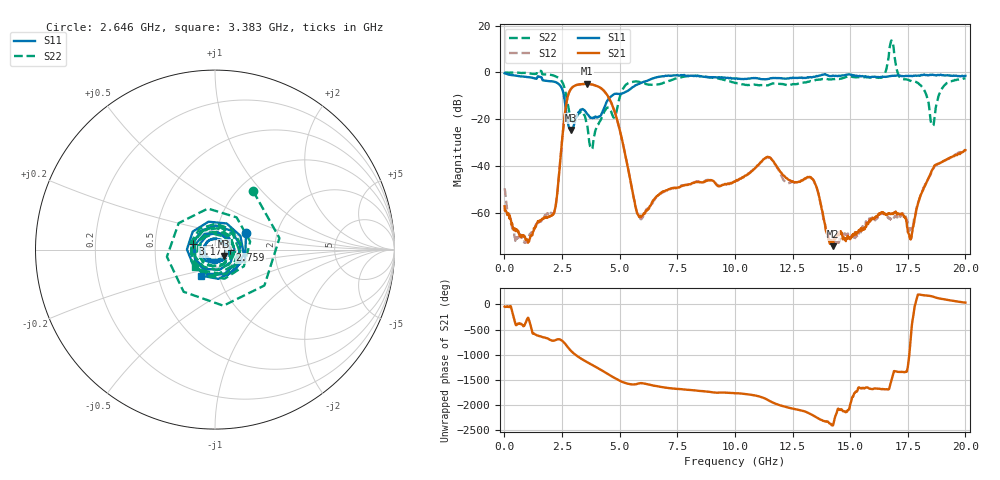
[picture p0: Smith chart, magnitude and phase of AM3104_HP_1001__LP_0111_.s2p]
!Created with skrf (http://scikit-rf.org).
# Hz S RI R 50.0
!freq ReS11 ImS11 ReS21 ImS21 ReS12 ImS12 ReS22 ImS22
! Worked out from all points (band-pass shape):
!   1601 points, 10 MHz to 20 GHz, reference 50 ohm
!   highest |S21| = -4.87 dB at 3.571 GHz (marker M1); lowest = -74.1 dB at 14.25 GHz (marker M2)
!   |S21| within 3 dB of the highest: 2.836 GHz to 4.32 GHz (1.484 GHz wide, 41.5 % of centre)
!   lowest |S11| = -24.6 dB at 2.884 GHz (marker M3), VSWR 1.13, Z = 54.9 - j3.83 ohm
!   |S11| at or under -10 dB: 2.583 GHz to 4.658 GHz (2.075 GHz wide, 57.3 % of centre)
!   |S22| runs from -32.6 to 13.6 dB; largest |S21 - S12| = 0.037
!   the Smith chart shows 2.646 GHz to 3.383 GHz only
!   S11 on the Smith chart (normalised r, x): 2.646 GHz: 1.39, +0.27; 2.759 GHz: 1.18, -0.01; 3.171 GHz: 0.78, +0.05; 3.383 GHz: 0.82, -0.24
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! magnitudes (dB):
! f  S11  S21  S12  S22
! 10 MHz  -0.3  -57.1  -49.4  0.0
! 884.6 MHz  -1.8  -70.1  -72.6  -0.2
! 2.121 GHz  -3.9  -60.6  -60.1  -1.3
! 2.646 GHz  -14.1  -16.0  -16.0  -8.2
! 2.759 GHz  -21.5  -10.0  -10.0  -13.9
! 2.884 GHz  -24.6  -7.1  -7.2  -19.9
! 3.171 GHz  -17.9  -5.3  -5.3  -18.1
! 3.346 GHz  -15.8  -5.0  -5.1  -16.5
! 3.383 GHz  -15.6  -5.0  -5.0  -16.7
! 3.571 GHz  -17.4  -4.9  -4.9  -21.8
! 3.771 GHz  -19.3  -5.1  -5.1  -31.9
! 4.695 GHz  -9.7  -14.3  -14.4  -18.5
! 5.845 GHz  -4.9  -61.7  -61.9  -4.0
! 6.682 GHz  -1.9  -52.4  -52.4  -5.1
! 10.01 GHz  -2.7  -46.6  -46.7  -4.5
! 11.44 GHz  -2.8  -36.1  -36.2  -5.5
! 13.34 GHz  -2.1  -45.3  -45.3  -3.7
! 14.25 GHz  -1.3  -74.1  -72.3  -2.9
! 16.68 GHz  -1.6  -60.5  -62.3  7.2
! 17.61 GHz  -1.5  -70.8  -66.5  -3.5
! 18.56 GHz  -0.9  -41.5  -41.8  -22.3
! 20 GHz  -1.5  -33.2  -33.1  -2.6
